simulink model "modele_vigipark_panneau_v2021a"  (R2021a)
settings: Solver=ode15s  StartTime=0.0  StopTime=10  RelTol=1e-3  EnableMultiTasking=on
libraries: nesl_utility x4, fl_lib x3, ee_lib x2

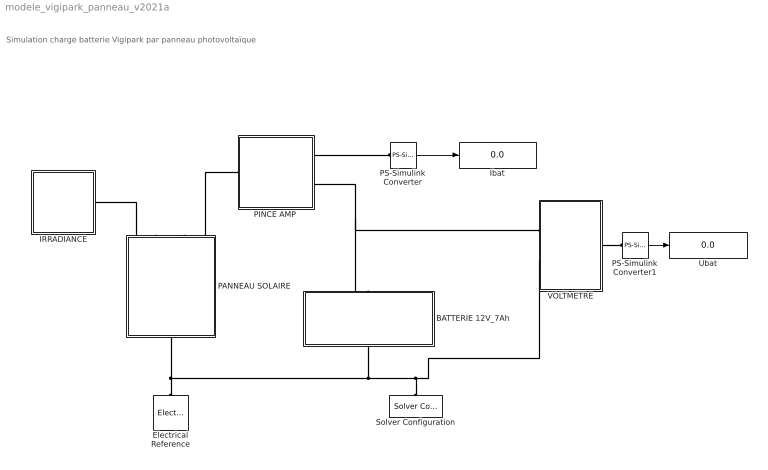
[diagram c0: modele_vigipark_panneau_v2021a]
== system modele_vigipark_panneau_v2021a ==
  note: Simulation charge batterie Vigipark par panneau photovoltaïque
  BATTERIE 12V_7Ah : Subsystem
  Electrical Reference : fl_lib/Electrical/Electrical Elements/Electrical Reference
  IRRADIANCE : Subsystem  mask{IRR=250}
      mask prompts: IRR "Irradiance (w/m2)"
  Ibat : Display
  PANNEAU SOLAIRE : Subsystem  mask{temp=25}
      mask prompts: temp "temperature panneau °C"
  "PINCE AMP " : Subsystem
  PS-Simulink Converter : nesl_utility/PS-Simulink Converter  PhysicalDomain=network_engine_domain  SubClassName=ps_output  LeftPortType=input  RightPortType=output  PseudoPeriodic=off  Frequencies=[]  Unit=A  AffineConversion=off
  PS-Simulink Converter1 : nesl_utility/PS-Simulink Converter  PhysicalDomain=network_engine_domain  SubClassName=ps_output  LeftPortType=input  RightPortType=output  PseudoPeriodic=off  Frequencies=[]  Unit=V  AffineConversion=off
  Solver Configuration : nesl_utility/Solver Configuration  PhysicalDomain=network_engine_domain  SubClassName=solver  LeftPortType=input  RightPortType=generic  Tones=[]  Harmonics=[]  SimulateNoise=off  Profile=off  UseLocalSampling=off  EnableSwitchedLinearOptims=on  FrequencyDomain=off  UseCCode=off  RelTol=0.001  AbsTol=1e-06  MinStep=1e-09  ToWorkspace=off  RevertToSquareIcSolve=off  NumHomotopyIterations=100  PhasorMode=off  PhasorModeNumHarmonics=1  DoDC=off  ResidualTolerance=1e-9  UseLocalSolver=off  LocalSolverChoice=NE_BACKWARD_EULER_ADVANCER  LocalSolverSampleTime=.001  DoFixedCost=off  MaxNonlinIter=3  MaxModeIter=2  ComputeImpulses=off  ImpulseIterations=2  LinearAlgebra=Sparse  EquationFormulation=NE_TIME_EF  DelaysMemoryBudget=1024  AutomaticFiltering=on  FilteringTimeConstant=0.001  PartitionStorageMethod=AS_NEEDED  PartitionMemoryBudget=1024  PartitionMethod=FAST
  Ubat : Display
  VOLTMETRE : Subsystem
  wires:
  PS-Simulink Converter/1 -> Ibat/1
  PS-Simulink Converter1/1 -> Ubat/1
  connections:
  "PINCE AMP "/RConn2 -- BATTERIE 12V_7Ah/LConn1 -- VOLTMETRE/RConn1
  Solver Configuration/RConn1 -- PANNEAU SOLAIRE/LConn1 -- Electrical Reference/LConn1 -- BATTERIE 12V_7Ah/RConn1 -- VOLTMETRE/RConn2
  IRRADIANCE/LConn1 -- PANNEAU SOLAIRE/RConn1
  "PINCE AMP "/RConn1 -- PS-Simulink Converter/LConn1
  "PINCE AMP "/LConn1 -- PANNEAU SOLAIRE/RConn2
  VOLTMETRE/LConn1 -- PS-Simulink Converter1/LConn1

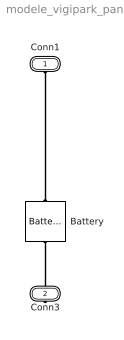
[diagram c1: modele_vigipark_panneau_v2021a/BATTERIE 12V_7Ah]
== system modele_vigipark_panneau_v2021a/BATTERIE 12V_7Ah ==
  Battery : ee_lib/Sources/Battery  Vnom=12 V  prm_dir=1  R1_dis=2 Ohm  R1_ch=2 Ohm  R1=0.0018 Ohm  prm_AH=2  AH=7 hr*A  V1=11.5 V  AH1=3.5 hr*A  prm_R2=1  R2=2000 Ohm  prm_dyn=1  Rp1=0.005 Ohm  tau1=30 s  Rp2=0.005 Ohm  tau2=30 s  Rp3=0.005 Ohm  tau3=30 s  Rp4=0.005 Ohm  tau4=30 s  Rp5=0.005 Ohm  tau5=30 s  prm_fade=1  N_fade=100  AH_fade=45 hr*A  R1_fade=2.02 Ohm  R1_ch_fade=2.02 Ohm  V1_fade=10.35 V  prm_age=1  prm_age_OCV=1  OCV_age=0.9  SOC_age=60  Tmeas_age=298.15 K  delta_time_age_vec=[0] d  temperature_age_vec=[273] K  OCV_scaling_age=2.2134e6  OCV_offset_age=1.632e6  temp_exp_age=0.515833569 V  t_exp_age=0.75  i_specify=off  i_priority=None  i=0 A  i_nominal_specify=off  i_nominal_unit=A  i_nominal_value=1  v_specify=off  v_priority=None  v=0 V  v_nominal_specify=off  v_nominal_unit=V  v_nominal_value=1  charge_specify=off  charge_priority=High  charge=50 hr*A  charge_nominal_specify=off  charge_nominal_unit=hr*A  charge_nominal_value=1  num_cycles_specify=off  num_cycles_priority=High  num_cycles=0  num_cycles_nominal_specify=off  num_cycles_nominal_unit=1  num_cycles_nominal_value=1  thermal_mass=30000 J/K  Tmeas=298.15 K  Vnom_T2=12 V  R1_T2=2.2 Ohm  R1_T2_dis=2.2 Ohm  R1_T2_ch=2.2 Ohm  V1_T2=11.4 V  R2_T2=2200 Ohm  Rp1_T2=0.005 Ohm  tau1_T2=30 s  Rp2_T2=0.005 Ohm  tau2_T2=30 s  Rp3_T2=0.005 Ohm  tau3_T2=30 s  Rp4_T2=0.005 Ohm  tau4_T2=30 s  Rp5_T2=0.005 Ohm  tau5_T2=30 s  Tmeas2=273.15 K  temperature_specify=off  temperature_priority=High  temperature=298.15 K  temperature_nominal_specify=off  temperature_nominal_unit=K  temperature_nominal_value=1
  Conn1 : PMIOPort  Side=Left
  Conn3 : PMIOPort  Port=2  Side=Right
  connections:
  Battery/RConn1 -- Conn3/RConn1
  Battery/LConn1 -- Conn1/RConn1

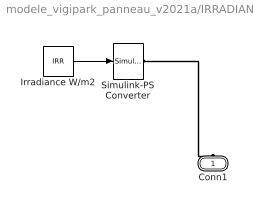
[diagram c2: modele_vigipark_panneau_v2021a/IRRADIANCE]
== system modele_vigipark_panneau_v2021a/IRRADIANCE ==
  Irradiance W/m2 : Constant  Value=IRR
  Simulink-PS Converter : nesl_utility/Simulink-PS Converter  PhysicalDomain=network_engine_domain  SubClassName=ps_input  LeftPortType=input  RightPortType=output  PseudoPeriodic=off  Frequencies=[]  NoiseDistribution=none  NoiseParameters=[]  Unit=1  AffineConversion=off  FilteringAndDerivatives=zero  SimscapeFilterOrder=1  InputFilterTimeConstant=.001  UdotUserProvided=1
  Conn1 : PMIOPort  Side=Left
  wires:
  Irradiance W/m2/1 -> Simulink-PS Converter/1
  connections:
  Simulink-PS Converter/RConn1 -- Conn1/RConn1

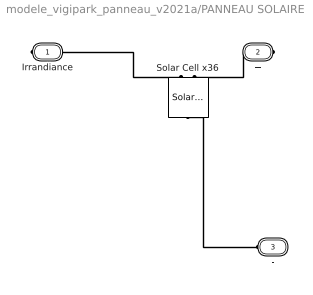
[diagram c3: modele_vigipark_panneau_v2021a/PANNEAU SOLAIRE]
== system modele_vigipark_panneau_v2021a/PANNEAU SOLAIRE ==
  Solar Cell x36 : ee_lib/Sources/Solar Cell  prm=1  Isc=0.7 A  Voc=0.569444 V  Is=1e-6 A  Is2=0 A  Iph=7.34 A  Ir0=1000 W/m^2  ec=1.5  N2=2  Rs=0 Ohm  Rp=Inf Ohm  N_series=36  TIPH1=0 1/K  EG=1.11 eV  TXIS1=3  TXIS2=3  TRS1=0  TRP1=0  Tmeas=25 degC  TFIXED=temp degC  thermal_mass=100 J/K  initial_temperature=25 degC
  Irrandiance : PMIOPort  Tag=PMCPort  Side=Right
  + : PMIOPort  Tag=PMCPort  Port=2  Side=Right
  - : PMIOPort  Tag=PMCPort  Port=3  Side=Left
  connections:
  Irrandiance/RConn1 -- Solar Cell x36/LConn1
  +/RConn1 -- Solar Cell x36/LConn2
  -/RConn1 -- Solar Cell x36/RConn1

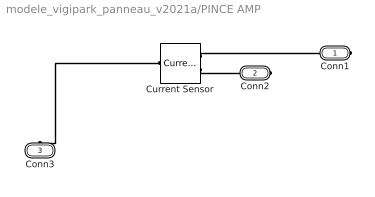
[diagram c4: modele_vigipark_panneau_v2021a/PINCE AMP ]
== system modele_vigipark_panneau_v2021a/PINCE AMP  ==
  Current Sensor : fl_lib/Electrical/Electrical Sensors/Current Sensor
  Conn1 : PMIOPort  Side=Right
  Conn2 : PMIOPort  Port=2  Side=Right
  Conn3 : PMIOPort  Port=3  Side=Left
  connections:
  Current Sensor/LConn1 -- Conn3/RConn1
  Current Sensor/RConn1 -- Conn1/RConn1
  Current Sensor/RConn2 -- Conn2/RConn1

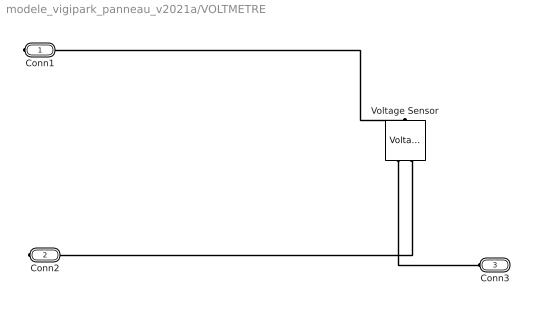
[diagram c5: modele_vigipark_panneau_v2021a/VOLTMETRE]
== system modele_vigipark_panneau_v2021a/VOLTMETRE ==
  Voltage Sensor : fl_lib/Electrical/Electrical Sensors/Voltage Sensor
  Conn1 : PMIOPort  Side=Right
  Conn2 : PMIOPort  Port=2  Side=Right
  Conn3 : PMIOPort  Port=3  Side=Left
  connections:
  Voltage Sensor/RConn1 -- Conn3/RConn1
  Conn1/RConn1 -- Voltage Sensor/LConn1
  Voltage Sensor/RConn2 -- Conn2/RConn1
